PROGRAM MAIN
VAR CONSTANT	
	// single-channel usage
    cInitSource				: ST_MA_MultiArray_InitPars := ( eTypeCode := eMA_TypeCode_LREAL, nDims := 1, aDimSizes := [cBufferLength]);
	// multi-channel usage
	//cInitSource				: ST_MA_MultiArray_InitPars := ( eTypeCode := eMA_TypeCode_LREAL, nDims := 2, aDimSizes := [cChannels, cBufferLength]);	
END_VAR
VAR
	nInputSelection			: UDINT := 1;						// Switch between hardware and function generator	
	nSample					: UDINT;
	nWindow					: UDINT;
	nChannel				: UDINT;
	aEl3632 AT %I*			: ARRAY[1..cOversamples] OF INT;	// Input from hardware e.g. EL3632
                        	
	aBufferSignal			: ARRAY [1..cOversamples] OF LREAL;  // signal part
	aBufferSignalSum		: ARRAY [1..cOversamples] OF LREAL;  // signal part 
	aBufferNoise			: ARRAY [1..cOversamples] OF LREAL;  // signal noise
	aBuffer					: ARRAY [1..cChannels] OF ARRAY [1..cOversamples] OF LREAL;  // aBufferNoise + aBufferSignal + ... 
					    	
	fbSource				: FB_CMA_Source :=(	stInitPars := cInitSource, nOwnID := eID_Source, aDestIDs := [eID_Spectrum]);
	fbSinkSpectrum			: FB_CMA_Sink := (nOwnID := eID_SinkSpectrum);
	fbSinkStatistics		: FB_CMA_Sink := (nOwnID := eID_SinkStatistics);
	
	aSignalGenerator		: ARRAY [1..cChannels] OF ARRAY [1..cMaxWindows] OF FB_FunctionGenerator;	// Signal generator
	bInitSignalGenerator	: BOOL := TRUE;
	aSetFrequency			: ARRAY [1..cChannels] OF ARRAY [1..cMaxWindows] OF LREAL;		// Hz
	aSetAmplitude			: ARRAY [1..cMaxWindows] OF LREAL;								// peak amplitude of sine signal
	fFrequencyShift			: LREAL := 420.0;
	fbNoiseGenerator		: FB_NoiseGenerator();				// Noise generator
	aNoiseParams			: ARRAY [1..2] OF LREAL := [0,2];	// mean,stddev
	
	aSpectrumResult			: ARRAY [1..cChannels] OF ARRAY [1..cFFTResult] OF LREAL;					// Copy of result
	aStatisticsResult		: ARRAY [1..cChannels] OF ARRAY[1..cMaxWindows] OF ARRAY[1..8] OF LREAL;	// Copy of result
	nCountResults			: ULINT;
		
	fbErrHist				: FB_HRErrHist; 					// error monitoring
END_VAR

CASE nInputSelection OF
	0:  (* input from EL3632 *)
		FOR nChannel := 1 TO cChannels DO
			FOR nSample := 1 TO cOversamples DO
				aBuffer[nChannel][nSample] := INT_TO_LREAL(aEl3632[nSample]);
			END_FOR
		END_FOR
		
	1:  (* signal generator *)
		IF bInitSignalGenerator THEN
			bInitSignalGenerator := FALSE;
			FOR nChannel := 1 TO cChannels DO
				FOR nWindow := 1 TO cMaxWindows DO
					aSetFrequency[nChannel][nWindow] := 100.0 + (nWindow-1) * 1080 + (nChannel-1) * fFrequencyShift;
					aSetAmplitude[nWindow] := 2.4 + nWindow * 4.2;
				END_FOR
			END_FOR
		END_IF
	
		fbNoiseGenerator(	bEnable		:= TRUE,
							aParam 		:= aNoiseParams,
							aSignal		:= aBufferNoise);
		FOR nChannel := 1 TO cChannels DO	
			FOR nSample := 1 TO cOversamples DO
				aBuffer[nChannel][nSample] := aBufferNoise[nSample];
			END_FOR
		END_FOR
		
		FOR nChannel := 1 TO cChannels DO
			FOR nSample := 1 TO cOversamples DO
				aBufferSignalSum[nSample] := 0;
			END_FOR
			FOR nWindow := 1 TO cMaxWindows DO
				aSignalGenerator[nChannel][nWindow] (	fFrequency 	:= aSetFrequency[nChannel][nWindow],
														fAmplitude 	:= aSetAmplitude[nWindow],
														eFunction 	:= E_FunctionType.Sine,
														aSignal		:= aBufferSignal );
				FOR nSample := 1 TO cOversamples DO
					aBufferSignalSum[nSample] := aBufferSignalSum[nSample] + aBufferSignal[nSample];
				END_FOR
			END_FOR
			FOR nSample := 1 TO cOversamples DO
				aBuffer[nChannel][nSample] := aBuffer[nChannel][nSample] + aBufferSignalSum[nSample];
			END_FOR
		END_FOR
END_CASE					

// Call source to collect data; use Input2DStd for multi-channel usage
fbSource.Input1DStd( pDataIn 		:= ADR(aBuffer),
					 nDataInSize 	:= SIZEOF(aBuffer), 
					 eElementType 	:= eMA_TypeCode_LREAL,
					 nOptionPars	:= cCMA_Option_MarkInterruption ); 
IF fbSource.bError THEN
	fbErrHist.AddError(bErr:=TRUE, hrErrCode:=fbSource.hrErrorCode, sErrSource:='MAIN.fbSource'); // error monitoring
	// ToDo: if error
END_IF

// Push results to sink; use Output2DStd for multi-channel usage
fbSinkSpectrum.Output1DStd(	pDataOut 		:= ADR(aSpectrumResult), 
							nDataOutSize 	:= SIZEOF(aSpectrumResult), 
							eElementType 	:= eMA_TypeCode_LREAL, 
							nOptionPars		:= 0);
IF fbSinkSpectrum.bError THEN
	fbErrHist.AddError(bErr:=TRUE, hrErrCode:=fbSinkSpectrum.hrErrorCode, sErrSource:='MAIN.fbSinkSpectrum'); // error monitoring
	// ToDo: if error
END_IF

// Push results to sink; use Output3DStd for multi-channel usage
fbSinkStatistics.Output2DStd(	pDataOut 		:= ADR(aStatisticsResult), 
								nDataOutSize 	:= SIZEOF(aStatisticsResult), 
								eElementType 	:= eMA_TypeCode_LREAL, 
								nOptionPars		:= 0);
IF fbSinkStatistics.bError THEN
	fbErrHist.AddError(bErr:=TRUE, hrErrCode:=fbSinkStatistics.hrErrorCode, sErrSource:='MAIN.fbSinkStatistics'); // error monitoring
	// ToDo: if error
END_IF

END_PROGRAM
